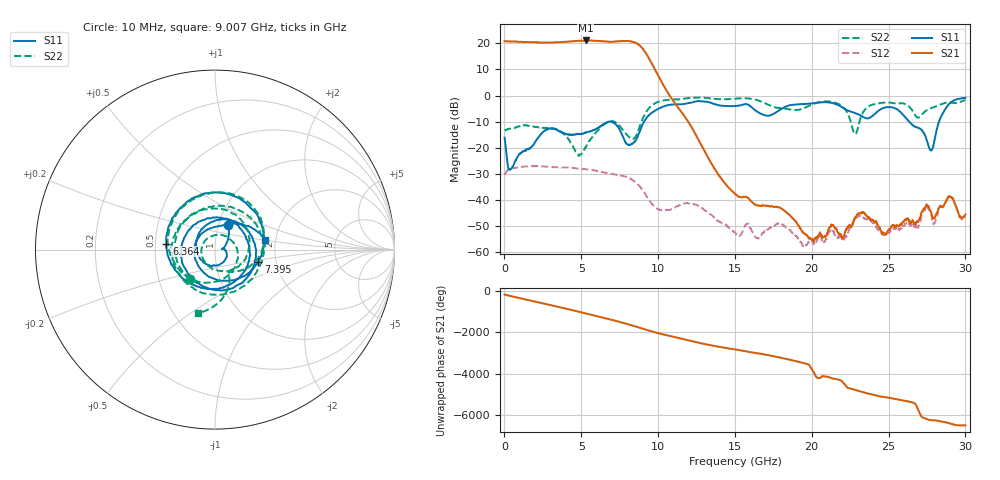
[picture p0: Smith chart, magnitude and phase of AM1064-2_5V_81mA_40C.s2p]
!Agilent	"Technologies,E8364B,MY43040894,A.07.50.67"
!Agilent	E8364B:	A.07.50.67
!Date:	"Wednesday,"	May	"01,"	2019	6:25:38
!Correction:	S11(Full	2	"Port(1,2))"
!S21(Full	2	"Port(1,2))"
!S12(Full	2	"Port(1,2))"
!S22(Full	2	"Port(1,2))"
!S2P	File:	Measurements:	"S11,"	"S21,"	"S12,"	S22:
#	Hz	S	dB	R	50
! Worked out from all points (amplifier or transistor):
!   1601 points, 10 MHz to 30 GHz, reference 50 ohm
!   highest |S21| = 21.1 dB at 5.277 GHz (marker M1)
!   |S21| within 3 dB of that: start of sweep to 8.97 GHz
!   unconditionally stable (mu >= 1): start of sweep to end of sweep
!   at 4.996 GHz: K = 1.31, MAG = 21.2 dB, |S12| = -28.0 dB
!   at 15.01 GHz: K = 2270.93, MAG = -29.2 dB, |S12| = -52.4 dB
!   at 30 GHz: K = 1148.57, MAG = -33.2 dB, |S12| = -46.4 dB
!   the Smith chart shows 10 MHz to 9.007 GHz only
!   S11 on the Smith chart (normalised r, x): 10 MHz: 1.11, +0.32; 6.364 GHz: 0.57, +0.04; 7.395 GHz: 1.62, -0.24; 9.007 GHz: 1.76, +0.21
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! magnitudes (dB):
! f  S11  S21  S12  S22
! 10 MHz  -16.1  20.8  -30.4  -13.4
! 403.6 MHz  -28.1  20.7  -28.0  -12.6
! 2.728 GHz  -13.1  20.3  -27.2  -12.4
! 5.015 GHz  -14.6  21.0  -28.0  -22.3
! 5.277 GHz  -14.0  21.1  -28.1  -19.9
! 6.364 GHz  -11.3  20.8  -29.2  -11.5
! 7.395 GHz  -12.0  20.8  -30.4  -11.1
! 8.145 GHz  -18.9  20.8  -31.6  -16.0
! 9.007 GHz  -10.9  17.9  -36.2  -8.7
! 10.02 GHz  -5.0  7.5  -43.5  -2.4
! 12.46 GHz  -2.2  -15.1  -41.7  -0.8
! 15.01 GHz  -4.0  -37.6  -52.4  -1.2
! 17.95 GHz  -5.4  -42.9  -48.8  -4.8
! 20.01 GHz  -3.0  -55.3  -55.5  -3.4
! 21.87 GHz  -4.1  -53.0  -53.6  -3.6
! 22.82 GHz  -6.7  -46.6  -47.1  -14.7
! 23.59 GHz  -8.7  -46.1  -47.4  -4.5
! 25.01 GHz  -4.4  -51.2  -52.3  -2.7
! 26.91 GHz  -12.2  -48.4  -50.6  -8.4
! 27.77 GHz  -21.0  -44.5  -45.5  -4.8
! 29.03 GHz  -2.7  -38.7  -38.5  -2.7
! 30 GHz  -0.8  -45.5  -46.4  -1.7
